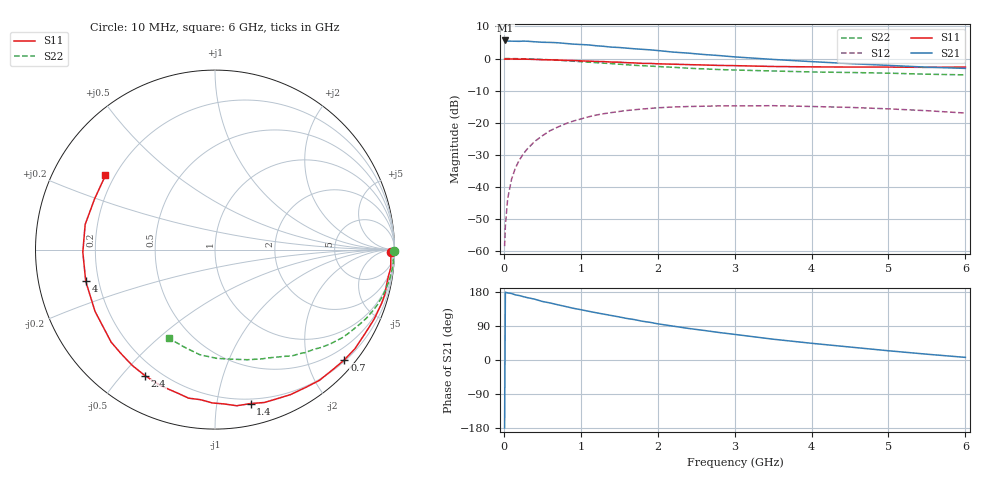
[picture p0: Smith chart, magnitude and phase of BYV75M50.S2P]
! SIEMENS Small Signal Semiconductors
! BFY420
! Si NPN RF SIEGET Grounded Emitter Transistor in MICRO-X
! VCE = 0.75 V  IC = 0.5 mA
! Common Emitter S-Parameters:  October  1996
# GHz  S  MA  R  50
!  f  S11  S21  S12  S22
! GHz  MAG  ANG  MAG  ANG  MAG  ANG  MAG  ANG
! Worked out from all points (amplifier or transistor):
!   36 points, 10 MHz to 6 GHz, reference 50 ohm
!   highest |S21| = 5.6 dB at 20 MHz (marker M1)
!   |S21| within 3 dB of that: start of sweep to 1.936 GHz
!   unconditionally stable (mu >= 1): 4.74 GHz to end of sweep
!   at 250 MHz: K = 0.04, MSG = 17.6 dB, |S12| = -29.8 dB
!   at 1.4 GHz: K = 0.23, MSG = 10.2 dB, |S12| = -16.8 dB
!   at 6 GHz: K = 1.37, MAG = 3.3 dB, |S12| = -17.0 dB
!   S11 on the Smith chart (normalised r, x): 10 MHz: 72, -43; 700 MHz: 0.23, -2.70; 1.4 GHz: 0.16, -1.24; 2.4 GHz: 0.15, -0.58; 4 GHz: 0.15, -0.12; 6 GHz: 0.17, +0.30
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0.01  0.9797 -0.7  1.902 -179.3  0.0012 88.1  0.999 -0.3
0.02  0.9801 -1.3  1.911 178.8  0.0025 88.3  0.9999 -0.6
0.05  0.9809 -3.0  1.867 177.1  0.0066 87.5  0.9989 -1.5
0.1  0.9844 -5.9  1.863 175.5  0.0132 86.8  0.9946 -3.2
0.15  0.9773 -8.7  1.858 171.9  0.0197 83.6  0.9962 -4.9
0.2  0.976 -12.0  1.851 170.1  0.0261 82.4  0.9933 -6.4
0.3  0.9759 -17.6  1.86 164.8  0.0386 78.6  0.9874 -9.6
0.4  0.968 -23.5  1.823 160.6  0.0511 74.4  0.9782 -12.7
0.5  0.958 -29.2  1.791 154.5  0.0627 70.7  0.9673 -15.8
0.7  0.9471 -40.4  1.76 145.8  0.0856 63.2  0.941 -21.6
0.9  0.9322 -51.4  1.676 136.6  0.1061 55.6  0.9091 -27.0
1.1  0.9109 -62.5  1.63 128.7  0.1237 49.0  0.8777 -32.1
1.4  0.8803 -77.0  1.504 117.3  0.1441 39.5  0.8325 -38.9
1.8  0.8403 -95.4  1.391 102.3  0.1637 28.5  0.7738 -46.7
2.2  0.8166 -111.7  1.26 89.4  0.176 18.7  0.7311 -54.1
2.4  0.8037 -118.9  1.213 83.3  0.1791 14.9  0.7066 -57.4
2.8  0.781 -132.1  1.112 72.5  0.1831 7.1  0.6734 -63.6
3.5  0.7518 -152.8  0.968 54.9  0.1844 -3.8  0.6396 -73.6
4  0.7415 -166.2  0.895 44.1  0.1793 -10.5  0.6178 -81.2
4.5  0.7366 -178.9  0.833 34.2  0.1735 -16.6  0.6062 -89.0
5.5  0.728 157.0  0.734 15.3  0.1541 -25.7  0.5698 -107.3
6  0.7372 145.9  0.702 6.9  0.1417 -28.2  0.5569 -117.4
